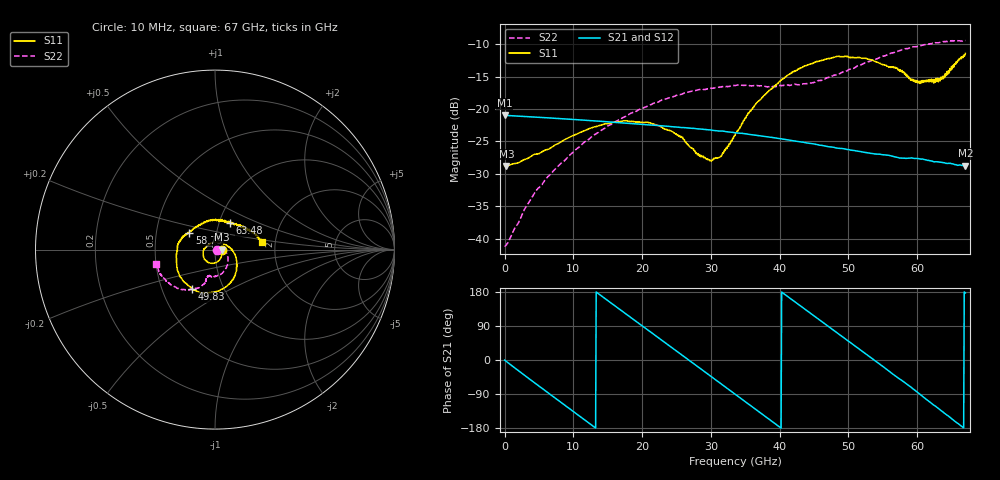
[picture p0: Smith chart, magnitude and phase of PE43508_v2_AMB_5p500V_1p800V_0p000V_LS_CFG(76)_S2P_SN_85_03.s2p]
!Keysight Technologies,N5227A,US51270237,A.10.43.00
!Date: Wednesday, August 22, 2018 17:14:33
!Correction: S11(Full 2 Port(1,3))
!S31(Full 2 Port(1,3))
!S13(Full 2 Port(1,3))
!S33(Full 2 Port(1,3))
!S2P File: Measurements: S11, S31, S13, S33:
# Hz S  dB  R 50
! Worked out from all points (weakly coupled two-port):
!   801 points, 10 MHz to 67 GHz, reference 50 ohm
!   highest |S21| = -20.97 dB at 10 MHz (marker M1); lowest = -28.7 dB at 67 GHz (marker M2)
!   lowest |S11| = -28.8 dB at 261.2 MHz (marker M3), VSWR 1.08, Z = 53.8 - j0.107 ohm
!   |S11| at or under -10 dB: start of sweep to end of sweep
!   |S22| runs from -41.1 to -9.4 dB; largest |S21 - S12| = 0.00053
!   S11 on the Smith chart (normalised r, x): 10 MHz: 1.08, -0.00; 49.83 GHz: 0.71, -0.34; 58.79 GHz: 0.74, +0.14; 63.48 GHz: 1.13, +0.34; 67 GHz: 1.71, +0.15
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1e7  -28.74 -0.7  -20.97 -0.2  -20.97 -0.2  -41.07 -1.1
2.612125e8  -28.80 -1.6  -21.00 -3.8  -21.00 -3.8  -40.97 6.4
4.615562e9  -26.95 -28.4  -21.26 -63.6  -21.27 -63.6  -32.55 24.6
1.123082e10  -23.49 -74.0  -21.70 -152.7  -21.71 -152.7  -25.48 -4.4
1.74274e10  -21.84 -115.2  -22.16 124.6  -22.16 124.6  -21.21 -33.3
2.236791e10  -22.56 -150.9  -22.57 58.7  -22.56 58.7  -18.89 -54.5
2.571741e10  -24.34 176.7  -22.86 14.3  -22.85 14.2  -17.75 -67.4
2.81458e10  -26.88 140.8  -23.06 -18.3  -23.07 -18.3  -17.05 -76.0
2.982055e10  -27.94 106.7  -23.21 -40.7  -23.21 -40.7  -16.83 -82.0
3.14953e10  -27.19 66.0  -23.39 -62.9  -23.39 -62.9  -16.62 -87.7
3.3505e10  -24.09 27.2  -23.65 -90.1  -23.66 -90.1  -16.37 -93.6
3.55147e10  -20.64 -0.1  -23.90 -117.0  -23.91 -116.9  -16.37 -97.6
3.836178e10  -17.30 -27.9  -24.32 -154.9  -24.33 -154.8  -16.57 -102.8
4.137632e10  -14.70 -53.5  -24.77 164.7  -24.78 164.8  -16.37 -104.7
4.472582e10  -13.01 -80.6  -25.33 120.1  -25.32 120.1  -15.99 -105.5
4.983381e10  -11.88 -119.6  -26.24 52.1  -26.22 52.1  -14.08 -107.4
5.276462e10  -12.31 -145.3  -26.75 12.7  -26.73 12.6  -12.74 -113.0
5.586291e10  -13.59 -178.0  -27.13 -29.0  -27.12 -29.5  -11.53 -122.4
5.879372e10  -15.32 146.5  -27.58 -67.6  -27.59 -67.9  -10.65 -132.3
6.130585e10  -15.82 102.4  -27.86 -103.6  -27.86 -104.0  -10.04 -142.1
6.348302e10  -15.40 60.4  -28.21 -133.6  -28.26 -134.3  -9.70 -151.2
6.7e10  -11.46 9.0  -28.71 177.0  -28.79 176.9  -9.46 -166.0
